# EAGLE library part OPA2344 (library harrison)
OP AMP
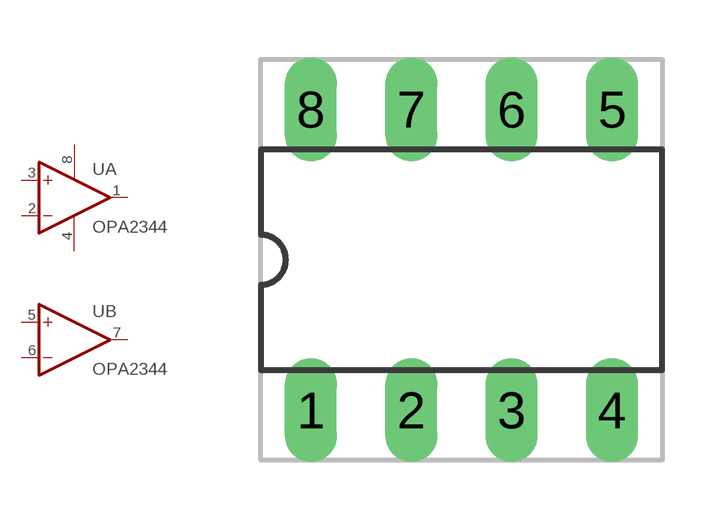
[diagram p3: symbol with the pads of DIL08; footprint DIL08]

Designator prefix U; gates A=OPAMP B=OPAMP P=PWR+-

## OPA2344  [DIL08]
1  A:OUT  out
2  A:-IN  in
3  A:+IN  in
4  P:V-  pwr
5  B:+IN  in
6  B:-IN  in
7  B:OUT  out
8  P:V+  pwr

## Footprint DIL08 (pad centres in mm)
drill 0.813 long: 1 -3.81,-3.81; 2 -1.27,-3.81; 3 1.27,-3.81; 4 3.81,-3.81; 5 3.81,3.81; 6 1.27,3.81; 7 -1.27,3.81; 8 -3.81,3.81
